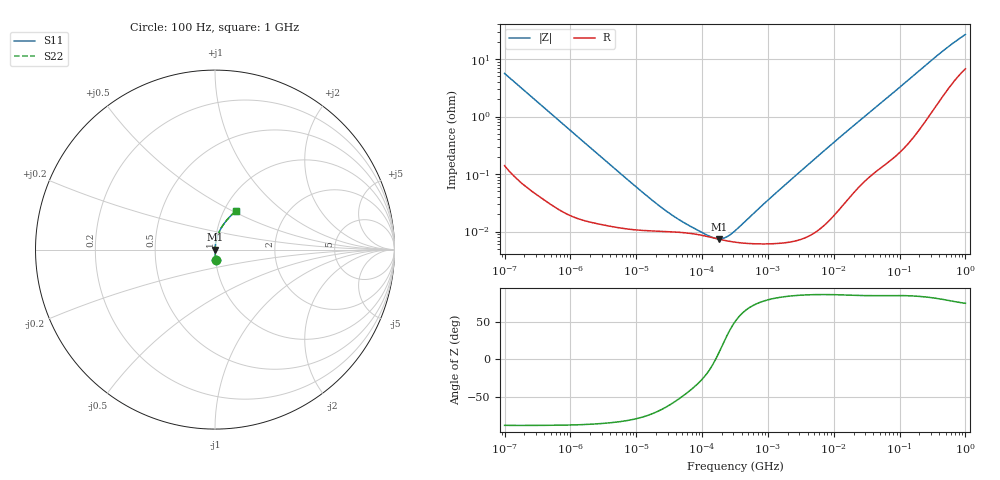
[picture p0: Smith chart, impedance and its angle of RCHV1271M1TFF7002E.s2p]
! RCHV1271M1TFF7002E  S-PARAMETER MODEL  (AEC-Q200 qualified)
! Model Generated by ELNA Corporation (http://www.ty-top.com)
! Version 1.0
! ELNA Control No. 240229
! Copyright (c) 2024 ELNA CO.,LTD. All Rights Reserved.
! Products Name : CONDUCTIVE POLYMER HYBRID ALUMINUM ELECTROLYTIC CAPACITORS
! Characteristics :
!  Capacitance  :  270uF  ,  Rated voltage  :  25V
!  Operating Temp. Range  :  -55 to +105 degC  ,  Endurance  :  10000hr at 105 degC
!  Dimension D  :  10mm  ,  Dimension L  :  8.7mm
! Frequency Range : 100Hz - 1GHz
! External Node Assignments :
!  1  o---| |---o  2
# MHz S RI R 50
!Freq[MHz].  S11 Real  S11 Imag  S21 Real  S21 Imag  S12 Real  S12 Imag  S22 Real  S22 Imag
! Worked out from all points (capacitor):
!   401 points, 100 Hz to 1 GHz, reference 50 ohm
!   read as one part in series: C = 283 uF near 108 Hz
!   lowest |Z| = 7.48 mohm at 179.9 kHz (marker M1)
!   series resonance near 160.4 kHz, so ESL is about 3.5 nH
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0.0001  0.00453 -0.0558  0.9955 0.0558  0.9955 0.0558  0.00453 -0.0558
0.000113  0.00365 -0.0495  0.9963 0.0495  0.9963 0.0495  0.00365 -0.0495
0.000309  0.00077 -0.0183  0.9992 0.0183  0.9992 0.0183  0.00077 -0.0183
0.001488  0.000175 -0.00386  0.9998 0.00386  0.9998 0.00386  0.000175 -0.00386
0.009495  0.000108 -0.000617  0.9999 0.000617  0.9999 0.000617  0.000108 -0.000617
0.022131  0.000102 -0.000265  0.9999 0.000265  0.9999 0.000265  0.000102 -0.000265
0.04217  9.78e-05 -0.000137  0.9999 0.000137  0.9999 0.000137  9.78e-05 -0.000137
0.087096  8.86e-05 -5.58e-05  0.9999 5.58e-05  0.9999 5.58e-05  8.86e-05 -5.58e-05
0.102329  8.55e-05 -4.13e-05  0.9999 4.13e-05  0.9999 4.13e-05  8.55e-05 -4.13e-05
0.179887  7.39e-05 1.16e-05  0.9999 -1.16e-05  0.9999 -1.16e-05  7.39e-05 1.16e-05
0.280221  6.68e-05 6.31e-05  0.9999 -6.31e-05  0.9999 -6.31e-05  6.68e-05 6.31e-05
0.316228  6.55e-05 7.96e-05  0.9999 -7.96e-05  0.9999 -7.96e-05  6.55e-05 7.96e-05
0.356862  6.43e-05 9.76e-05  0.9999 -9.76e-05  0.9999 -9.76e-05  6.43e-05 9.76e-05
1.059254  6.14e-05 0.000369  0.9999 -0.000369  0.9999 -0.000369  6.14e-05 0.000369
4.704354  9.25e-05 0.00168  0.9999 -0.00168  0.9999 -0.00168  9.25e-05 0.00168
15.13561  0.000353 0.0053  0.9996 -0.0053  0.9996 -0.0053  0.000353 0.0053
69.9842  0.00217 0.0226  0.9978 -0.0226  0.9978 -0.0226  0.00217 0.0226
176.8072  0.00796 0.0553  0.992 -0.0553  0.992 -0.0553  0.00796 0.0553
395.8221  0.0312 0.1145  0.9688 -0.1145  0.9688 -0.1145  0.0312 0.1145
668.3439  0.0699 0.1691  0.9301 -0.1691  0.9301 -0.1691  0.0699 0.1691
922.5714  0.1052 0.2053  0.8948 -0.2053  0.8948 -0.2053  0.1052 0.2053
1000  0.1153 0.2145  0.8847 -0.2145  0.8847 -0.2145  0.1153 0.2145
